{attribute 'qualified_only'}
{attribute 'strict'}
TYPE E_DirectControlState :
(
	Ready:=0,
	WaitForActivationTime:=1,
	PerformTest:=2,
	WaitForExecution:=3,
	WaitForChange:=4,
	MirrorBlockedCommand:=5
);
END_TYPE
